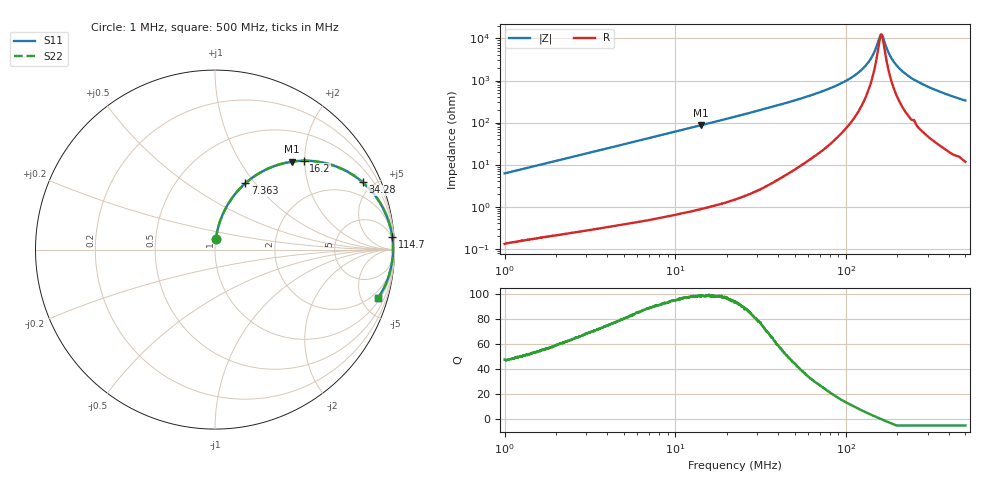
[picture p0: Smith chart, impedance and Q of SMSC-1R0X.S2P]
!s-Parameter Generated by FASTRON Sdn. Bhd.
!FASTRON P/N : SMSC-1R0X
!Keysight Technologies,E4991B,MY54100416,A.01.15
!Date: Thu Mar 19 09:51:41 2026
!Version  : Rev00 Thu Mar 19 09:51:41 2026
!Data & Calibration Information:
!PortZ  Port1:50+j0  Port2:50+j0
!When reading, reference impedance value at option line is always used.
! Remarks : This data is being provided solely for informational purposes.
!Freq	S11	S21	S12	S22
# Hz S dB R 50
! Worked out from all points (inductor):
!   1601 points, 1 MHz to 500 MHz, reference 50 ohm
!   read as one part in series: L = 979 nH near 1.032 MHz
!   highest Q = 98.7 at 14.19 MHz (marker M1), where L = 971 nH
!   self-resonance near 160.8 MHz
!   S11 on the Smith chart (normalised r, x): 1 MHz: 1.00, +0.12; 7.363 MHz: 1.01, +0.90; 16.2 MHz: 1.02, +1.98; 34.28 MHz: 1.06, +4.35; 114.7 MHz: 4, +28; 500 MHz: 1.23, -6.67
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1000000  -24.22 85.3  -0.03 -3.5  -0.03 -3.5  -24.22 85.3
2820919  -15.43 79.4  -0.15 -9.7  -0.15 -9.7  -15.43 79.4
7362819  -7.81 65.4  -0.83 -24.0  -0.83 -24.0  -7.81 65.4
7957584  -7.26 63.7  -0.95 -25.7  -0.95 -25.7  -7.26 63.7
1.419459e7  -3.73 48.8  -2.47 -40.6  -2.47 -40.6  -3.73 48.8
1.619854e7  -3.10 45.0  -3.01 -44.4  -3.01 -44.4  -3.10 45.0
2.236068e7  -1.88 35.7  -4.67 -53.7  -4.67 -53.7  -1.88 35.7
3.427987e7  -0.88 24.5  -7.63 -64.6  -7.63 -64.6  -0.88 24.5
6.307767e7  -0.26 12.4  -13.37 -75.8  -13.37 -75.8  -0.26 12.4
8.912629e7  -0.13 7.3  -17.96 -79.5  -17.96 -79.5  -0.13 7.3
1.147233e8  -0.09 4.0  -23.05 -79.8  -23.05 -79.8  -0.09 4.0
1.27408e8  -0.08 2.7  -26.28 -78.0  -26.28 -78.0  -0.08 2.7
1.382358e8  -0.07 1.8  -29.90 -73.9  -29.90 -73.9  -0.07 1.8
1.459609e8  -0.07 1.1  -33.38 -67.1  -33.38 -67.1  -0.07 1.1
1.559241e8  -0.07 0.4  -39.76 -38.7  -39.76 -38.7  -0.07 0.4
1.596005e8  -0.07 0.1  -41.73 -11.6  -41.73 -11.6  -0.07 0.1
1.646376e8  -0.07 -0.3  -40.61 30.1  -40.61 30.1  -0.07 -0.3
1.77937e8  -0.07 -1.2  -33.09 67.2  -33.09 67.2  -0.07 -1.2
2.007053e8  -0.08 -2.6  -26.65 77.1  -26.65 77.1  -0.08 -2.6
2.418399e8  -0.11 -5.0  -21.21 79.1  -21.21 79.1  -0.11 -5.0
3.312556e8  -0.20 -9.3  -15.80 77.4  -15.80 77.4  -0.20 -9.3
5e8  -0.46 -16.5  -10.92 71.5  -10.92 71.5  -0.46 -16.5
